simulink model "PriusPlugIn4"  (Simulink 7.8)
settings: Solver=ode23t  StartTime=0.0  StopTime=1180  MaxStep=0.01  RelTol=1e-3
InitFcn:
  | init_Prius_GT
StopFcn:
  | Vyhodnoceni
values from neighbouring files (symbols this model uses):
  k = Nr/Ns    (= 2.6)    [init_Prius_GT.m]
  Mpr = Nr/(Nr+Ns)    (= 0.722222222222)    [init_Prius_GT.m]
  Mps = Ns/(Nr+Ns)    (= 0.277777777778)    [init_Prius_GT.m]
  om_diff_ic = 0    [init_Prius_GT.m]
  omric = 0    [init_Prius_GT.m]
  rpm_FMEP = [1,500,1000,1500,2000,2500,3000,3500,4000,4500,5000]    [init_Prius_GT.m]
  t_sample = 0.1    [init_Prius_GT.m]
  torque_FMEP = [0,0,0.58,0.66,0.75,0.84,0.93,1.1,1.3,1.4,1.5].*(Vdis/(4*pi))*100000    [init_Prius_GT.m]
  vf0 = 0    [init_Prius_GT.m]
undefined symbols (not defined in the file or in its folder): Battery, Battery_Pack, Clutch, Differential, Driveshaft, Engine, Environment, Gearbox, Motor, Powertrain, table_FMEP, Vehicle
libraries: simulink x24, simulink_extras x4, simulink_need_slupdate x1
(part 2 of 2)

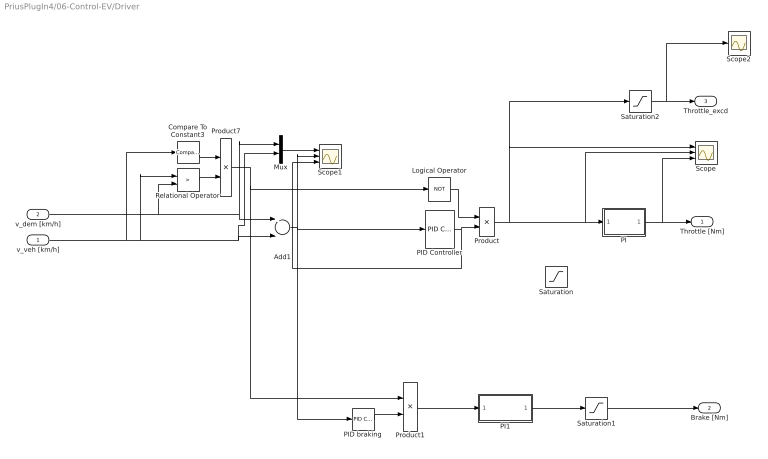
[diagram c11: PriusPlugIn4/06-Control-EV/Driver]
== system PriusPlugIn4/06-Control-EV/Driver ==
  v_veh [km/h] : Inport
  v_dem [km/h] : Inport  Port=2
  Add1 : Sum  Inputs=+-
  Compare To Constant3 : simulink/Logic and Bit Operations/Compare To Constant  relop=>  const=1  OutDataTypeStr=uint8  ZeroCross=off
  Logical Operator : Logic  Operator=NOT  AllPortsSameDT=off  OutDataTypeStr=boolean
  Mux : Mux  Inputs=2
  PI : Subsystem
  PI1 : Subsystem
  PID Controller : simulink/Continuous/PID Controller  Controller=PID  TimeDomain=Continuous-time  SampleTime=1  IntegratorMethod=Forward Euler  FilterMethod=Forward Euler  Form=Parallel  P=0.25  I=0.00015*6  D=0  N=100  InitialConditionSource=internal  InitialConditionForIntegrator=0  InitialConditionForFilter=0  ExternalReset=none  LimitOutput=on  UpperSaturationLimit=1.5  LowerSaturationLimit=0  LinearizeAsGain=off  AntiWindupMode=none  Kb=1  TrackingMode=off  Kt=1  PParamMin=[]  PParamMax=[]  IParamMin=[]  IParamMax=[]  DParamMin=[]  DParamMax=[]  NParamMin=[]  NParamMax=[]  KbParamMin=[]  KbParamMax=[]  KtParamMin=[]  KtParamMax=[]  POutMin=[]  POutMax=[]  IOutMin=[]  IOutMax=[]  DOutMin=[]  DOutMax=[]  NOutMin=[]  NOutMax=[]  KbOutMin=[]  KbOutMax=[]  KtOutMin=[]  KtOutMax=[]  IntegratorOutMin=[]  IntegratorOutMax=[]  FilterOutMin=[]  FilterOutMax=[]  SumOutMin=[]  SumOutMax=[]  SumI1OutMin=[]  SumI1OutMax=[]  SumI2OutMin=[]  SumI2OutMax=[]  SumI3OutMin=[]  SumI3OutMax=[]  SumDOutMin=[]  SumDOutMax=[]  SaturationOutMin=[]  SaturationOutMax=[]  IntegratorContinuousStateAttributes=''  IntegratorStateMustResolveToSignalObject=off  IntegratorRTWStateStorageClass=Auto  FilterContinuousStateAttributes=''  FilterStateMustResolveToSignalObject=off  FilterRTWStateStorageClass=Auto
  PID braking : simulink_need_slupdate/PID Controller  P=0.5  I=0.002  D=0
  Product : Product
  Product1 : Product
  Product7 : Product
  Relational Operator : RelationalOperator  Operator=>  OutDataTypeStr=boolean
  Saturation : Saturate  UpperLimit=1  LowerLimit=0
  Saturation1 : Saturate  UpperLimit=0  LowerLimit=-1
  Saturation2 : Saturate  UpperLimit=inf  LowerLimit=1
  Scope : Scope  NumInputPorts=3
  Scope1 : Scope  NumInputPorts=3
  Scope2 : Scope  NumInputPorts=3
  Throttle [Nm] : Outport
  Brake [Nm] : Outport  Port=2
  Throttle_excd : Outport  Port=3
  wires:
  PID braking/1 -> Product1/2
  Product1/1 -> PI1/1(In1)
  Add1/1 -> Scope1/2, PID braking/1, PID Controller/1
  v_dem [km/h]/1 -> Mux/1, Add1/1, Relational Operator/2
  v_veh [km/h]/1 -> Mux/2, Add1/2, Relational Operator/1, Compare To Constant3/1
  PID Controller/1 -> Scope1/3, Product/2
  Logical Operator/1 -> Product/1
  Saturation1/1 -> Brake [Nm]/1
  Product7/1 -> Product1/1, Logical Operator/1
  Compare To Constant3/1 -> Product7/1
  Relational Operator/1 -> Product7/2
  PI1/1(Out1) -> Saturation1/1
  Product/1 -> PI/1(In1), Scope/2, Scope/1, Saturation2/1
  Saturation2/1 -> Scope2/2, Throttle_excd/1
  Mux/1 -> Scope1/1
  PI/1(Out1) -> Throttle [Nm]/1, Scope/3

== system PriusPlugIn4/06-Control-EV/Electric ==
  v_veh : Inport
  SOC : Inport  Port=2
  Throttle : Inport  Port=3
  Compare To Constant : simulink/Logic and Bit Operations/Compare To Constant  relop=>=  const=30  OutDataTypeStr=uint8
  Compare To Constant2 : simulink/Logic and Bit Operations/Compare To Constant  relop=<  const=0.2  OutDataTypeStr=uint8
  Compare To Constant3 : simulink/Logic and Bit Operations/Compare To Constant  relop=>=  const=70  OutDataTypeStr=boolean
  Compare To Constant4 : simulink/Logic and Bit Operations/Compare To Constant  relop=<  const=65  OutDataTypeStr=boolean
  Constant : Constant
  Constant1 : Constant  Value=0
  Logical Operator : Logic  Inputs=3  AllPortsSameDT=off  OutDataTypeStr=boolean
  S-R Flip-Flop : simulink_extras/Flip Flops/S-R Flip-Flop  initial_condition=0
  Switch : Switch  Criteria=u2 > Threshold
  Out1 : Outport
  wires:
  S-R Flip-Flop/1 -> Logical Operator/1
  Compare To Constant/1 -> Logical Operator/2
  Logical Operator/1 -> Switch/2
  Constant/1 -> Switch/1
  Constant1/1 -> Switch/3
  Compare To Constant2/1 -> Logical Operator/3
  SOC/1 -> Compare To Constant/1
  Throttle/1 -> Compare To Constant2/1
  Switch/1 -> Out1/1  "Electric"
  v_veh/1 -> Compare To Constant3/1, Compare To Constant4/1
  Compare To Constant4/1 -> S-R Flip-Flop/1
  Compare To Constant3/1 -> S-R Flip-Flop/2

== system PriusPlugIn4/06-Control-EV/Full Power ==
  In1 : Inport
  SOC : Inport  Port=2
  Throttle : Inport  Port=3
  Brakes : Scope  NumInputPorts=5
  Compare To Constant : simulink/Logic and Bit Operations/Compare To Constant  relop=>=  const=0.99  OutDataTypeStr=boolean
  Compare To Constant1 : simulink/Logic and Bit Operations/Compare To Constant  relop=<  const=0.3  OutDataTypeStr=boolean
  Compare To Constant2 : simulink/Logic and Bit Operations/Compare To Constant  relop=>=  const=35  OutDataTypeStr=boolean
  Logical Operator : Logic  AllPortsSameDT=off  OutDataTypeStr=boolean
  S-R Flip-Flop : simulink_extras/Flip Flops/S-R Flip-Flop  initial_condition=0
  Out1 : Outport
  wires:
  Throttle/1 -> Compare To Constant/1, Compare To Constant1/1
  Compare To Constant/1 -> S-R Flip-Flop/1, Brakes/1
  Compare To Constant1/1 -> S-R Flip-Flop/2, Brakes/2
  S-R Flip-Flop/1 -> Logical Operator/1, Brakes/3  "Normal"
  SOC/1 -> Compare To Constant2/1
  Compare To Constant2/1 -> Logical Operator/2, Brakes/4
  Logical Operator/1 -> Out1/1, Brakes/5

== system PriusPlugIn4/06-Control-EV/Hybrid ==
  In1 : Inport
  SOC : Inport  Port=2
  Throttle : Inport  Port=3
  Compare To Constant1 : simulink/Logic and Bit Operations/Compare To Constant  relop=<=  const=65  OutDataTypeStr=boolean
  Compare To Constant2 : simulink/Logic and Bit Operations/Compare To Constant  relop=>=  const=70  OutDataTypeStr=boolean
  Compare To Constant3 : simulink/Logic and Bit Operations/Compare To Constant  relop=<=  const=30  OutDataTypeStr=uint8
  Compare To Constant4 : simulink/Logic and Bit Operations/Compare To Constant  relop=>  const=16  OutDataTypeStr=boolean
  Compare To Constant5 : simulink/Logic and Bit Operations/Compare To Constant  relop=>=  const=0.31  OutDataTypeStr=uint8
  Compare To Constant6 : simulink/Logic and Bit Operations/Compare To Constant  relop=>  const=16  OutDataTypeStr=boolean
  Constant2 : Constant
  Constant3 : Constant  Value=0
  Logical Operator : Logic  Operator=OR  AllPortsSameDT=off  OutDataTypeStr=boolean
  Logical Operator1 : Logic  AllPortsSameDT=off  OutDataTypeStr=boolean
  S-R Flip-Flop : simulink_extras/Flip Flops/S-R Flip-Flop  initial_condition=0
  Scope3 : Scope  NumInputPorts=3
  Switch1 : Switch  Criteria=u2 > Threshold
  Out1 : Outport
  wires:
  Constant2/1 -> Switch1/1
  Constant3/1 -> Switch1/3
  In1/1 -> Compare To Constant2/1, Compare To Constant1/1, Compare To Constant4/1
  SOC/1 -> Compare To Constant3/1
  Throttle/1 -> Compare To Constant5/1
  Switch1/1 -> Out1/1, Scope3/3  "Normal"
  Compare To Constant2/1 -> S-R Flip-Flop/1
  Compare To Constant1/1 -> S-R Flip-Flop/2
  Logical Operator/1 -> Switch1/2
  S-R Flip-Flop/1 -> Logical Operator/1, Scope3/1
  Compare To Constant5/1 -> Scope3/2, Logical Operator1/1
  Logical Operator1/1 -> Logical Operator/2
  Compare To Constant4/1 -> Logical Operator1/2

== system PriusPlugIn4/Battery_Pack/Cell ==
  Current [A] : Inport
  Charging : Subsystem
  Compare To Constant : simulink/Logic and Bit Operations/Compare To Constant  relop=>=  const=0  OutDataTypeStr=uint8
  Demux : Demux  Outputs=2
  Discharging : Subsystem
  Mux : Mux  Inputs=2
  Mux1 : Mux  Inputs=2
  SOC calculations Ah : Subsystem
  Switch : Switch
  Thermo-model : Subsystem
  U_terminal [V] : Outport
  P_loss [w] : Outport  Port=2
  SOC[%] : Outport  Port=3
  T_cell[C] : Outport  Port=4
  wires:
  Demux/2 -> Thermo-model/1(P_loss [W]), P_loss [w]/1
  Demux/1 -> U_terminal [V]/1
  Switch/1 -> Demux/1
  Discharging/2(P_loss[W]) -> Mux1/2
  Discharging/1(U_terminal [V]) -> Mux1/1
  Mux1/1 -> Switch/3
  Mux/1 -> Switch/1
  Compare To Constant/1 -> Switch/2
  Charging/2(P_loss[W]) -> Mux/2
  Charging/1(U_terminal [V]) -> Mux/1
  Thermo-model/1(T_cell[C]) -> T_cell[C]/1, Discharging/1(Temperature), Charging/1(Temperature)
  SOC calculations Ah/1(SOC) -> SOC[%]/1, Charging/2(SOC), Discharging/2(SOC)
  Current [A]/1 -> Discharging/3(Current_Cell [A]), Charging/3(Current_Cell [A]), SOC calculations Ah/1(Current [A]), Compare To Constant/1

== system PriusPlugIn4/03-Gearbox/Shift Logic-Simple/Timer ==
  Set : Inport
  Reset : Inport  Port=2
  Add1 : Sum  Inputs=-+
  Clock : Clock
  Memory : Memory
  S-R Flip-Flop : simulink_extras/Flip Flops/S-R Flip-Flop  initial_condition=0
  Switch1 : Switch  Threshold=1
  Terminator_1 : Terminator
  Count : Outport
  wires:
  S-R Flip-Flop/2 -> Terminator_1/1
  Reset/1 -> S-R Flip-Flop/2
  S-R Flip-Flop/1 -> Switch1/2
  Set/1 -> S-R Flip-Flop/1
  Add1/1 -> Count/1
  Clock/1 -> Switch1/3, Add1/2
  Memory/1 -> Switch1/1, Add1/1
  Switch1/1 -> Memory/1

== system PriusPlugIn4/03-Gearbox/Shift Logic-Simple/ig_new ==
  ig : Inport
  Trigger : TriggerPort
  Data Store Write1 : DataStoreWrite  DataStoreName=ig_new
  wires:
  ig/1 -> Data Store Write1/1

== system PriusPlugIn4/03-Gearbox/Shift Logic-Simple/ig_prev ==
  ig : Inport
  Trigger : TriggerPort
  Data Store Write1 : DataStoreWrite  DataStoreName=ig_prev
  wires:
  ig/1 -> Data Store Write1/1

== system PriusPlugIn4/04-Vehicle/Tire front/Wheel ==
  F_tire : Inport
  T_drsft : Inport  Port=2
  "        " : Gain  Gain=2*Vehicle.Tyre.Front.Rdyn
  " Inertia Wheel" : Gain  Gain=1/(2*Vehicle.Tyre.Rear.Inertia)
  Sum10 : Sum  Inputs=|-|+|
  "to Rot Speed     " : Integrator  InitialCondition=omric
  om_wheel : Outport
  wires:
  Sum10/1 -> " Inertia Wheel"/1
  " Inertia Wheel"/1 -> "to Rot Speed     "/1
  F_tire/1 -> "        "/1
  T_drsft/1 -> Sum10/2  "T_drv_sft"
  "        "/1 -> Sum10/1  "T_tire"
  "to Rot Speed     "/1 -> om_wheel/1  "om_wheel [rad/s]"

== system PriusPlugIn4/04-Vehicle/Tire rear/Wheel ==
  F_tire : Inport
  T_drsft : Inport  Port=2
  "        " : Gain  Gain=2*Vehicle.Tyre.Front.Rdyn
  " Inertia Wheel" : Gain  Gain=1/(2*Vehicle.Tyre.Front.Inertia)
  Sum10 : Sum  Inputs=|-|+|
  "to Rot Speed     " : Integrator  InitialCondition=omric
  om_wheel : Outport
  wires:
  "to Rot Speed     "/1 -> om_wheel/1  "om_wheel [rad/s]"
  "        "/1 -> Sum10/1  "T_tire"
  T_drsft/1 -> Sum10/2  "T_drv_sft"
  F_tire/1 -> "        "/1
  " Inertia Wheel"/1 -> "to Rot Speed     "/1
  Sum10/1 -> " Inertia Wheel"/1

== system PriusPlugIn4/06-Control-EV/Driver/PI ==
  In1 : Inport
  Add3 : Sum  Inputs=+-
  Constant : Constant  Value=10
  Integrator1 : Integrator
  Product1 : Product
  Out1 : Outport
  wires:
  Add3/1 -> Product1/1
  Product1/1 -> Integrator1/1
  In1/1 -> Add3/1
  Integrator1/1 -> Add3/2, Out1/1
  Constant/1 -> Product1/2

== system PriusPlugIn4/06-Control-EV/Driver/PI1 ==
  In1 : Inport
  Add3 : Sum  Inputs=+-
  Constant : Constant  Value=10
  Integrator1 : Integrator
  Product1 : Product
  Out1 : Outport
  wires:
  Constant/1 -> Product1/2
  Integrator1/1 -> Out1/1, Add3/2
  In1/1 -> Add3/1
  Product1/1 -> Integrator1/1
  Add3/1 -> Product1/1

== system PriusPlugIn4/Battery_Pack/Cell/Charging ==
  Temperature : Inport
  SOC : Inport  Port=2
  Current_Cell [A] : Inport  Port=3
  Add : Sum  Inputs=+-
  IR-Chrg : Lookup_n-D  BreakpointsForDimension1=Battery.Chrg.IR.Vektor_Temp  BreakpointsForDimension2=Battery.Chrg.IR.Vektor_SOC  Table=Battery.Chrg.IR.Data/1000  RndMeth=Simplest
  OCV-Chrg : Lookup_n-D  BreakpointsForDimension1=Battery.Chrg.OCV.Vektor_Temp  BreakpointsForDimension2=Battery.Chrg.OCV.Vektor_SOC  Table=Battery.Chrg.OCV.Data  RndMeth=Simplest
  Product : Product
  Product1 : Product
  U_terminal [V] : Outport
  P_loss[W] : Outport  Port=2
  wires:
  Product1/1 -> P_loss[W]/1
  Add/1 -> U_terminal [V]/1
  Product/1 -> Product1/1, Add/2
  Current_Cell [A]/1 -> Product1/2, Product/2
  IR-Chrg/1 -> Product/1
  OCV-Chrg/1 -> Add/1
  SOC/1 -> IR-Chrg/2, OCV-Chrg/2
  Temperature/1 -> IR-Chrg/1, OCV-Chrg/1

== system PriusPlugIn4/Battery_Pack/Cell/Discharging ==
  Temperature : Inport
  SOC : Inport  Port=2
  Current_Cell [A] : Inport  Port=3
  Add : Sum  Inputs=+-
  IR-Dchrg : Lookup_n-D  BreakpointsForDimension1=Battery.Dchrg.IR.Vektor_Temp  BreakpointsForDimension2=Battery.Dchrg.IR.Vektor_SOC  Table=Battery.Dchrg.IR.Data/1000  RndMeth=Simplest
  OCV-Dchrg : Lookup_n-D  BreakpointsForDimension1=Battery.Chrg.OCV.Vektor_Temp  BreakpointsForDimension2=Battery.Chrg.OCV.Vektor_SOC  Table=Battery.Chrg.OCV.Data  RndMeth=Simplest
  Product1 : Product
  Product2 : Product
  U_terminal [V] : Outport
  P_loss[W] : Outport  Port=2
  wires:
  OCV-Dchrg/1 -> Add/1
  Product2/1 -> P_loss[W]/1
  Add/1 -> U_terminal [V]/1
  Product1/1 -> Product2/1, Add/2
  Current_Cell [A]/1 -> Product2/2, Product1/2
  IR-Dchrg/1 -> Product1/1
  SOC/1 -> OCV-Dchrg/2, IR-Dchrg/2
  Temperature/1 -> OCV-Dchrg/1, IR-Dchrg/1

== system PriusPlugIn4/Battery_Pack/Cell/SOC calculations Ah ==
  Current [A] : Inport
  Add2 : Sum  Inputs=-+
  Capacity [Ah] : Constant  Value=6.5
  Divide2 : Product  Inputs=*/
  Gain1 : Gain  Gain=3600
  Gain2 : Gain  Gain=100
  Integrator1 : Integrator
  Product : Product
  SOCinit : Constant  Value=90/100
  Scope1 : Scope
  SOC : Outport
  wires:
  Add2/1 -> Divide2/1
  Divide2/1 -> Gain2/1
  Gain2/1 -> Scope1/1, SOC/1
  Product/1 -> Add2/2
  Integrator1/1 -> Add2/1
  SOCinit/1 -> Product/1
  Gain1/1 -> Product/2, Divide2/2
  Capacity [Ah]/1 -> Gain1/1
  Current [A]/1 -> Integrator1/1

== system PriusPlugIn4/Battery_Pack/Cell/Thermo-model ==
  P_loss [W] : Inport
  Temp : Constant  Value=30
  Terminator : Terminator
  T_cell[C] : Outport
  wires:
  P_loss [W]/1 -> Terminator/1
  Temp/1 -> T_cell[C]/1
